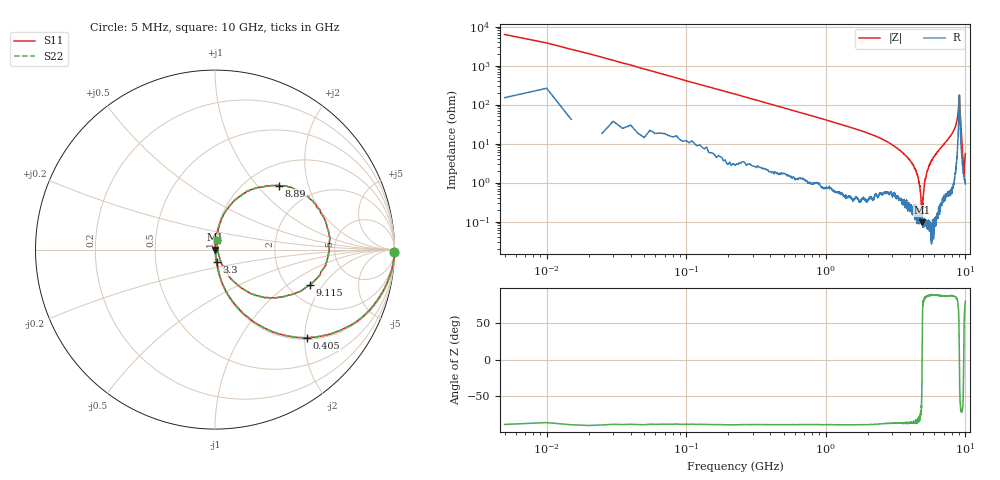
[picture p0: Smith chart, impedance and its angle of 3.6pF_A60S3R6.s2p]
! Amotech Co.,Ltd.
! http://www.amotech.co.kr/
! Part Number: A60S3R6
! These Parameters are Measured in Series Mode Connection
! Operation Temp=25[degC], DC Bias Voltage=0[V]
! Freq. Start=5[MHz] Stop=10[GHz], 2000[Steps]
! Date: Monday, July 13, 2020, 01:28:02
# GHZ S RI R 50.000000
!Freq.(Hz) S11(Real) S11(Imag) S21(Real) S21(Imag) S12(Real) S12(Imag) S22(Real) S22(Imag)
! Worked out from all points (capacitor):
!   2000 points, 5 MHz to 10 GHz, reference 50 ohm
!   read as one part in series: C = 3.87 pF near 55 MHz
!   lowest |Z| = 94.5 mohm at 4.89 GHz (marker M1)
!   series resonance near 4.897 GHz, so ESL is about 270 pH
!   S11 on the Smith chart (normalised r, x): 5 MHz: open; 405 MHz: 1.04, -2.05; 3.3 GHz: 1.01, -0.14; 8.89 GHz: 1.38, +1.32; 9.115 GHz: 2.60, -1.51; 10 GHz: 1.02, +0.11
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0.005  0.9994 -0.0159  0.000632 0.0159  0.000632 0.0159  0.9994 -0.0159
0.07  0.9671 -0.1636  0.0329 0.1636  0.0329 0.1636  0.9671 -0.1636
0.125  0.9091 -0.2737  0.0909 0.2737  0.0909 0.2737  0.9091 -0.2737
0.405  0.5128 -0.4907  0.4872 0.4907  0.4872 0.4907  0.5128 -0.4907
0.865  0.1872 -0.3798  0.8128 0.3798  0.8128 0.3798  0.1872 -0.3798
1.675  0.0539 -0.2169  0.9461 0.2169  0.9461 0.2169  0.0539 -0.2169
3.3  0.00933 -0.0706  0.9907 0.0706  0.9907 0.0706  0.00933 -0.0706
3.34  0.00865 -0.0684  0.9913 0.0684  0.9913 0.0684  0.00865 -0.0684
4.545  0.00135 -0.0152  0.9987 0.0152  0.9987 0.0152  0.00135 -0.0152
4.735  0.00109 -0.0068  0.9989 0.0068  0.9989 0.0068  0.00109 -0.0068
4.89  0.000924 -0.000192  0.9991 0.000192  0.9991 0.000192  0.000924 -0.000192
5.005  0.000863 0.00506  0.9991 -0.00506  0.9991 -0.00506  0.000863 0.00506
5.135  0.00108 0.0115  0.9989 -0.0115  0.9989 -0.0115  0.00108 0.0115
5.49  0.00167 0.0275  0.9983 -0.0275  0.9983 -0.0275  0.00167 0.0275
6.67  0.00882 0.0764  0.9912 -0.0764  0.9912 -0.0764  0.00882 0.0764
8.335  0.061 0.2166  0.939 -0.2166  0.939 -0.2166  0.061 0.2166
8.89  0.3577 0.3562  0.6423 -0.3562  0.6423 -0.3562  0.3577 0.3562
9.025  0.6248 0.1234  0.3752 -0.1234  0.3752 -0.1234  0.6248 0.1234
9.115  0.5277 -0.1978  0.4723 0.1978  0.4723 0.1978  0.5277 -0.1978
9.325  0.1092 -0.1819  0.8908 0.1819  0.8908 0.1819  0.1092 -0.1819
9.72  0.0161 -0.00266  0.9839 0.00266  0.9839 0.00266  0.0161 -0.00266
10  0.0121 0.0535  0.9879 -0.0535  0.9879 -0.0535  0.0121 0.0535
